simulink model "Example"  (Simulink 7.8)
settings: Solver=ode45  StartTime=0.0  StopTime=10.0  RelTol=1e-3
libraries: simulink x1

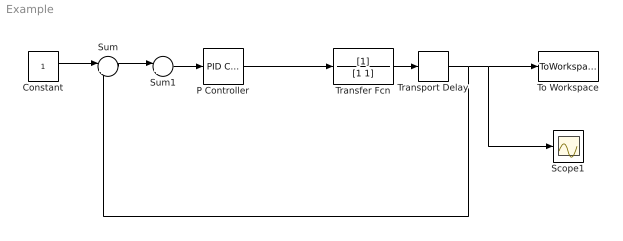
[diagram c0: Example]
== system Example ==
  Constant : Constant
  P Controller : simulink/Continuous/PID Controller  Controller=P  TimeDomain=Continuous-time  SampleTime=1  IntegratorMethod=Forward Euler  FilterMethod=Forward Euler  Form=Parallel  P=4  I=1  D=0  N=100  InitialConditionSource=internal  InitialConditionForIntegrator=0  InitialConditionForFilter=0  ExternalReset=none  LimitOutput=off  UpperSaturationLimit=inf  LowerSaturationLimit=-inf  LinearizeAsGain=off  AntiWindupMode=none  Kb=1  TrackingMode=off  Kt=1  PParamMin=[]  PParamMax=[]  IParamMin=[]  IParamMax=[]  DParamMin=[]  DParamMax=[]  NParamMin=[]  NParamMax=[]  KbParamMin=[]  KbParamMax=[]  KtParamMin=[]  KtParamMax=[]  POutMin=[]  POutMax=[]  IOutMin=[]  IOutMax=[]  DOutMin=[]  DOutMax=[]  NOutMin=[]  NOutMax=[]  KbOutMin=[]  KbOutMax=[]  KtOutMin=[]  KtOutMax=[]  IntegratorOutMin=[]  IntegratorOutMax=[]  FilterOutMin=[]  FilterOutMax=[]  SumOutMin=[]  SumOutMax=[]  SumI1OutMin=[]  SumI1OutMax=[]  SumI2OutMin=[]  SumI2OutMax=[]  SumI3OutMin=[]  SumI3OutMax=[]  SumDOutMin=[]  SumDOutMax=[]  SaturationOutMin=[]  SaturationOutMax=[]  IntegratorContinuousStateAttributes=''  IntegratorStateMustResolveToSignalObject=off  IntegratorRTWStateStorageClass=Auto  FilterContinuousStateAttributes=''  FilterStateMustResolveToSignalObject=off  FilterRTWStateStorageClass=Auto
  Scope1 : Scope
  Sum : Sum  Inputs=|+-
  Sum1 : Sum  Inputs=|+-
  To Workspace : ToWorkspace  VariableName=simout  SampleTime=-1  SaveFormat=Structure
  Transfer Fcn : TransferFcn  Denominator=[1 1]
  Transport Delay : TransportDelay
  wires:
  Constant/1 -> Sum/1
  Sum/1 -> Sum1/1
  Sum1/1 -> P Controller/1
  P Controller/1 -> Transfer Fcn/1
  Transfer Fcn/1 -> Transport Delay/1
  Transport Delay/1 -> Sum/2, To Workspace/1, Scope1/1
